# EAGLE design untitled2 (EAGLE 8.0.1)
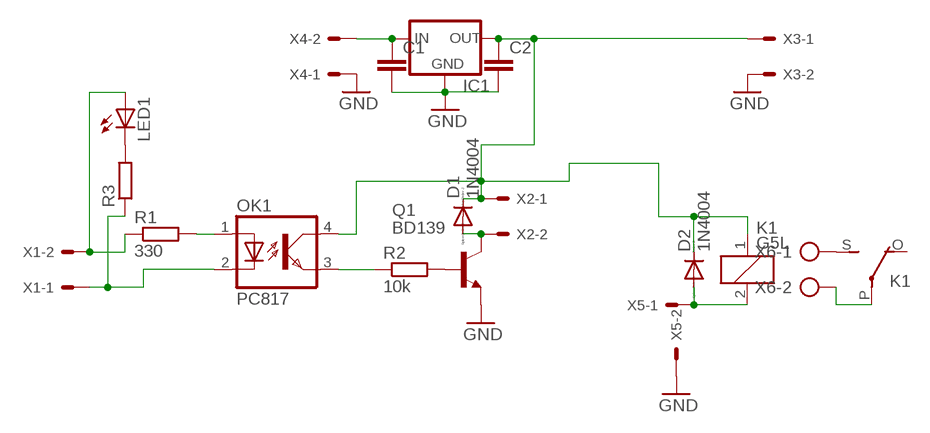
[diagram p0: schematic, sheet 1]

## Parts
C1  C-EU050-024X044  [C050-024X044]
C2  C-EU050-024X044  [C050-024X044]
D1  1N4004  [DO41-10]
D2  1N4004  [DO41-10]
IC1  78XXL  [78XXL]
K1  G5L  [G5LE]
LED1  LED3MM  [LED3MM]
OK1  PC817  [DIL04]
Q1  BD139  [TO126]
R1  330  R-EU_0207/7  [0207/7]
R2  10k  R-EU_0207/10  [0207/10]
R3  R-EU_0207/10  [0207/10]
X1  KK-156-2  [KK-156-2]
X2  KK-156-2  [KK-156-2]
X3  KK-156-2  [KK-156-2]
X4  KK-156-2  [KK-156-2]
X5  KK-156-2  [KK-156-2]
X6  AK300/2  [AK300/2]

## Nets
GND: C1.2 C2.2 IC1.GND Q1.1(E) X3.2 X4.1 X5.2
N$2: OK1.1(A) R1.2
N$3: OK1.2(C) R3.1 X1.1
N$4: Q1.3(B) R2.2
N$5: OK1.3(EMIT) R2.1
N$6: D1.A Q1.2(C) X2.2
N$8: C1.1 IC1.IN X4.2
N$10: C2.1 D1.C D2.C IC1.OUT K1.1 OK1.4(COL) X2.1 X3.1
N$12: D2.A K1.2 X5.1
N$13: K1.S(2:S) X6.1
N$14: K1.P(2:P) X6.2
N$19: LED1.K(C) R3.2
N$42: LED1.A R1.1 X1.2
Unconnected: K1.O(2:O)

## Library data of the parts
C1 C2 = resistor:C-EU: CAPACITOR, European symbol
D1 D2 = diode:1N4004: DIODE
IC1 = v-reg:78XXL: VOLTAGE REGULATOR
K1 = relay:G5L: RELAY 1 x switch, 10 A/120 V AC, 8 A/30 V ADC, Omron; OC_FARNELL: unknown; OC_NEWARK: unknown
LED1 = led:LED: LED
OK1 = optocoupler:PC817: SHARP OPTO COUPLER; MPN: PC817X4J000F; OC_FARNELL: 9707727; OC_NEWARK: 97K7059
Q1 = transistor-npn:BD139*: NPN Transistor
R1-R3 = resistor:R-EU_: RESISTOR, European symbol
X1-X5 = con-molex:KK-156-2: KK 156 HEADER; OC_FARNELL: unknown; OC_NEWARK: unknown
X6 = con-ptr500:AK300/2: CONNECTOR; OC_FARNELL: unknown; OC_NEWARK: unknown

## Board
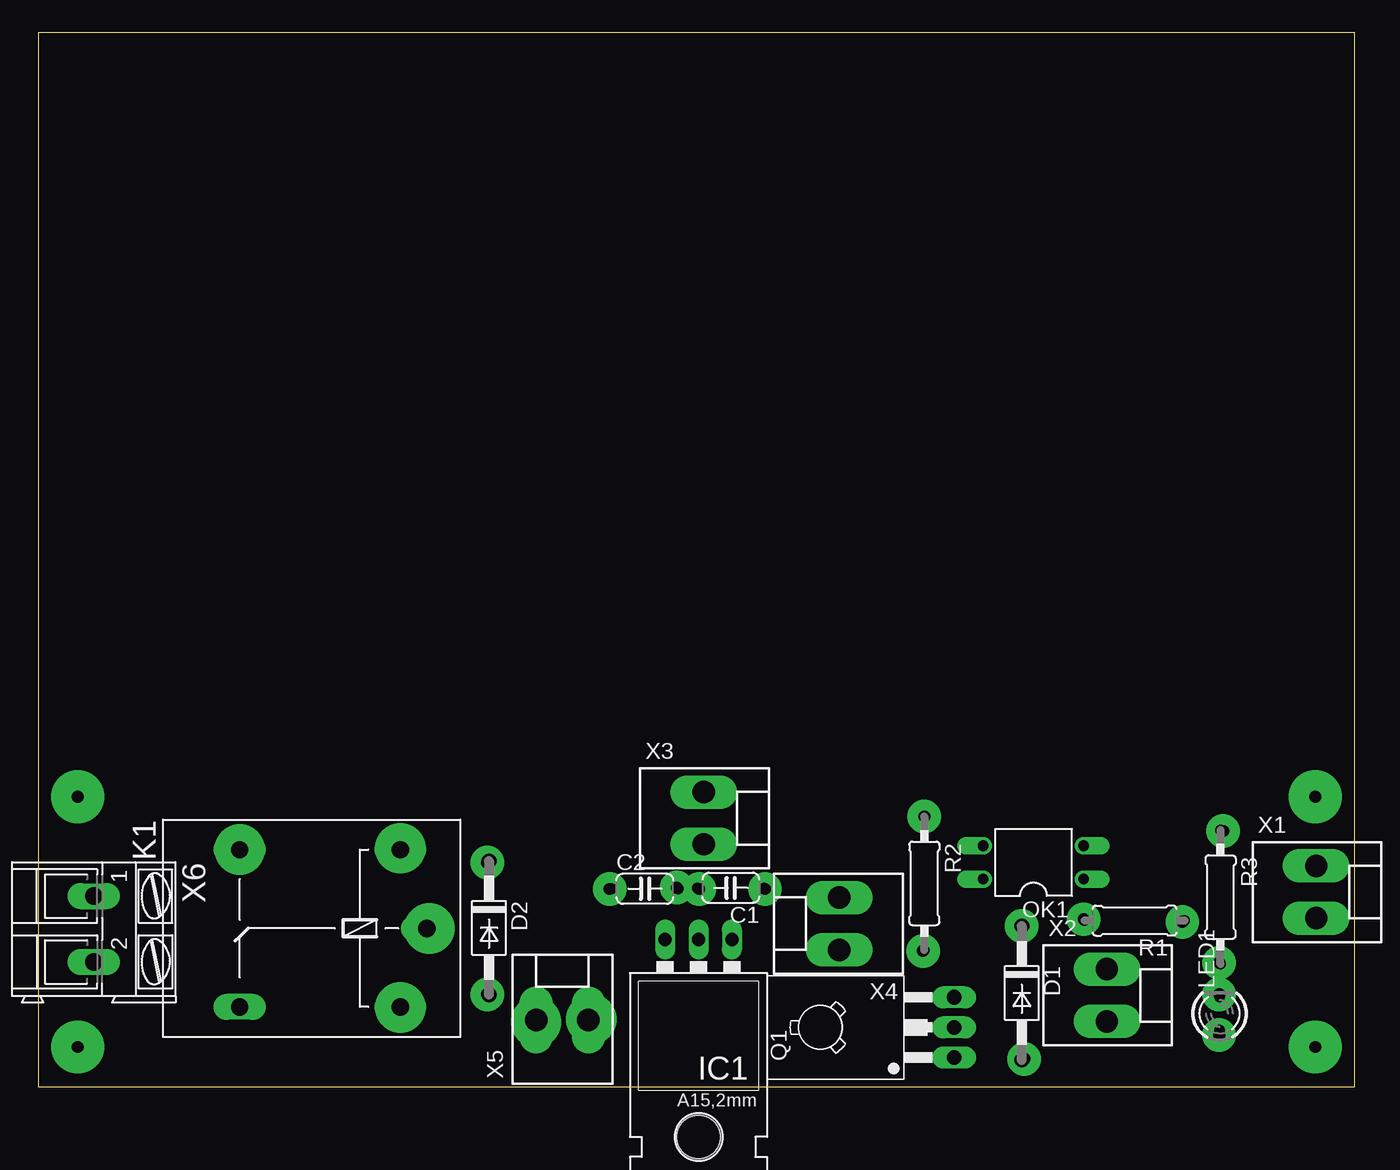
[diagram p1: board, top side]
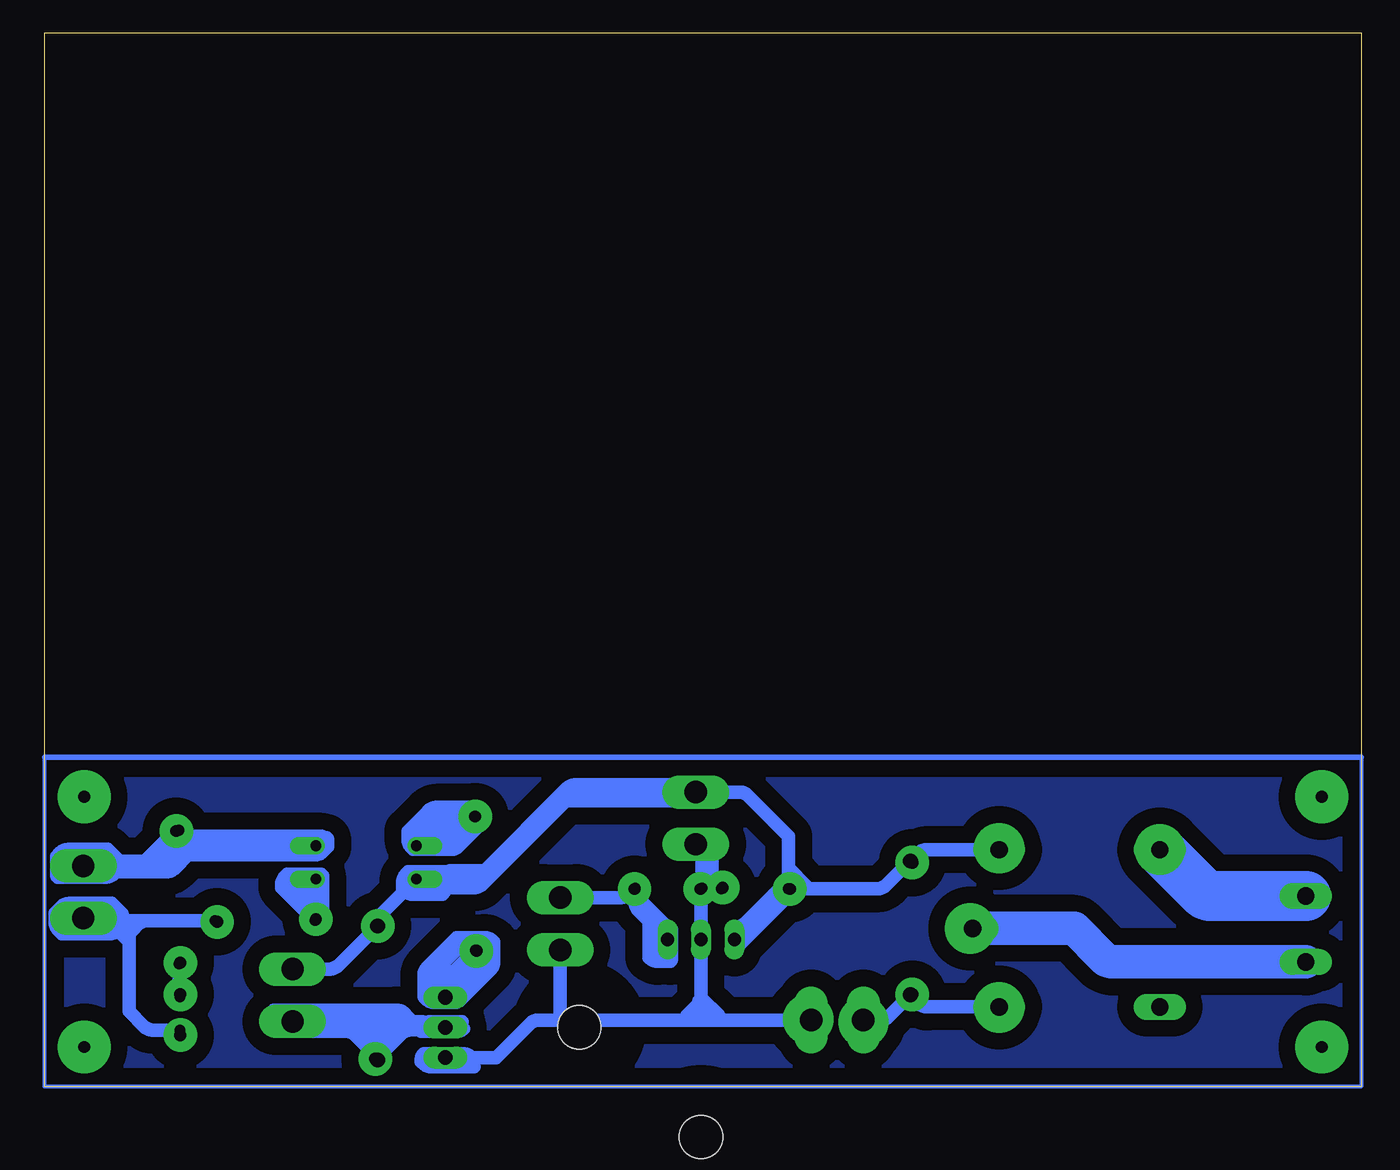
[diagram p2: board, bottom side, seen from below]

Size 100 x 80 mm. Coordinates in mm from the lower left corner, seen from the top.
Outline: 0,0 100,0 100,80 0,80 0,0
Copper layers (1*16): Top 0.035mm / dielectric 1.5mm / Bottom 0.035mm
Design rules "default": minimum track width 10mil, minimum drill 24mil, track to track 8mil, track to pad 8mil, pad to pad 8mil, via to via 8mil, smd to smd 8mil, copper to edge 40mil, drill to drill 8mil, minimum pad ring 10mil, minimum via ring 8mil, stop-mask expansion 4mil, vias tented up to drill 0mil, thermal gap 10mil

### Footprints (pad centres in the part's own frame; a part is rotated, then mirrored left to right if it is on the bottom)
C050-024X044 = drill 0.813 octagon: 1 -2.54,0; 2 2.54,0
DO41-10 = drill 1.118: A 5.08,0; C -5.08,0
78XXL = drill 1.016 long: GND 0,-3.81; IN -2.54,-3.81; OUT 2.54,-3.81 | hole 3.302: 0,11.176
G5LE = drill 1.321 long: 1 -7.493,-5.969; 2 -7.493,5.969; O 4.699,5.969; P -9.525,0; S 4.699,-5.969
LED3MM = drill 0.813 octagon: A -1.27,0; K 1.27,0
DIL04 = drill 0.813 offset: 1 -1.27,-3.81; 2 1.27,-3.81; 3 1.27,3.81; 4 -1.27,3.81
TO126 = drill 1.118 long: 1 -2.286,-5.08; 2 0,-5.08; 3 2.286,-5.08 | hole 3.302: 0,5.08
0207/7 = drill 0.813 octagon: 1 -3.81,0; 2 3.81,0
0207/10 = drill 0.813 octagon: 1 -5.08,0; 2 5.08,0
KK-156-2 = drill 1.7 pad 2.184 long: 1 -1.98,0; 2 1.98,0
AK300/2 = drill 1.321 long: 1 -2.515,0; 2 2.489,0

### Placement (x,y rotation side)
C1  52.61,15.08 180 top
C2  46.07,15.02 0 top
D1  74.71,7.1 270 top
D2  34.24,12.05 270 top
IC1  50.15,7.35 180 top
K1  20,12.01 180 top
LED1  89.73,5.55 90 top
OK1  75.59,17.02 90 top
Q1  64.48,4.49 90 top
R1  83.27,12.6 180 top
R2  67.3,15.43 270 top
R3  89.8,14.38 270 top
X1  97.07,14.77 270 top
X2  81.17,6.93 270 top
X3  50.55,20.38 270 top
X4  60.85,12.36 90 top
X5  39.8,5.05 0 top
X6  4.21,11.95 270 top

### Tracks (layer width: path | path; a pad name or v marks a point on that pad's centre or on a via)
GND
  Bottom 1.016: 50,5.05 X5.2 | 60.7,5.05 50,5.05 | 60.7,5.05 62.44,5.05 arc-45 63.14,4.76 65.7,2.2 Q1.1 arc45 Q1.1 | 50,5.05 arc45 50.15,5.41 IC1.GND 50.15,14.89 arc45 C1.2 | C2.2 49.92,15.02 arc45 C1.2 | C1.2 50.07,17.51 arc-45 50.36,18.21 X3.2 | X4.1 60.85,5.41 arc-45 60.7,5.05
N$1
  pour Bottom (isolate 1.27): 1,24 99,24 99,1 1,1
N$2
  Bottom 1.016: OK1.1 79.4,12.74 arc45 R1.2
N$3
  Bottom 1.016: X1.1 92.92,16.75 arc-45 92.22,17.04 R3.1 88.92,18.58 arc-45 88.22,18.29 OK1.2
N$4
  Bottom 1.016: Q1.3 69.56,7.68 arc45 69.27,8.38 R2.2
N$5
  Bottom 1.016: R2.1 69.68,20.51 arc-45 70.38,20.22 71.5,19.1 71.5,18.97 arc45 OK1.3
N$6
  Bottom 1.016: 74.9,4.49 Q1.2 | 74.9,4.49 81.48,4.49 arc45 81.5,4.5 arc45 81.42,4.71 X2.2 | D1.A 74.71,4.03 arc-45 74.9,4.49
N$7
  Bottom 0.305: 0,25 0,0 100,0 100,25
  Bottom 0.406: 0,25 100,25
N$8
  Bottom 1.016: X4.2 56.3,14.34 arc-45 55.6,14.63 C1.1 55.15,14.03 arc-45 54.86,13.33 IC1.IN
N$9  (via drill 0.9 pad 2.54)
  other vias: 34.1,17
N$10
  Bottom 1.016: K1.1 32.98,17.98 arc-45 33.68,17.69 D2.C 36.06,15.31 arc45 36.76,15.02 C2.1 43.92,14.62 | IC1.OUT arc-45 47.23,11.32 43.92,14.62 | 43.92,14.62 43.79,14.76 arc-45 43.5,15.46 43.5,19 46.57,22.07 arc-45 47.27,22.36 X3.1 60.13,22.36 arc-45 60.83,22.07 67.1,15.8 71.66,15.8 arc-45 OK1.4 74.42,13.11 arc-45 74.71,12.41 D1.C 77.69,9.2 arc45 78.39,8.91 X2.1
N$11  (via drill 0.9 pad 2.54)
  other vias: 34.1,7
N$12
  Bottom 1.016: X5.1 36.57,5.05 arc-45 35.87,5.34 D2.A 33.6,6.33 arc-45 32.9,6.04 K1.2
N$13
  Bottom 3.81: X6.1 11.37,14.46 arc45 12.08,14.76 K1.S
N$14
  Bottom 2.54: X6.2 18.85,9.46 arc45 19.55,9.75 21.8,12 29.5,12 arc45 K1.P
N$15  (via drill 0.9 pad 2.54)
  other vias: 43.4,15
N$16  (via drill 0.9 pad 2.54)
  other vias: 48.5,15.1
N$17  (via drill 0.9 pad 2.54)
  other vias: 50.2,15
N$18  (via drill 0.9 pad 2.54)
  other vias: 55.2,15
N$19
  Bottom 1.016: R3.2 89.8,6.99 arc-45 LED1.K
N$20  (via drill 0.9 pad 2.54)
  other vias: 67.2,10.3
N$21  (via drill 0.9 pad 2.54)
  other vias: 74.7,12.2
N$22  (via drill 0.9 pad 2.54)
  other vias: 74.9,2.1
N$23  (via drill 0.9 pad 2.54)
  other vias: 79.4,12.7
N$24  (via drill 0.9 pad 2.54)
  other vias: 86.9,12.5
N$25  (via drill 0.9 pad 2.54)
  other vias: 89.7,9.4
N$26  (via drill 0.9 pad 2.54)
  other vias: 89.7,7
N$27  (via drill 0.9 pad 2.54)
  other vias: 89.7,3.9
N$28  (via drill 0.9 pad 2.54)
  other vias: 90,19.4
N$29  (via drill 0.9 pad 2.54)
  other vias: 67.3,20.5
N$30  (via drill 0.9 pad 3.81)
  other vias: 27.5,6
N$31  (via drill 0.9 pad 3.81)
  other vias: 29.7,12
N$32  (via drill 0.9 pad 3.81)
  other vias: 27.5,18.1
N$33  (via drill 0.9 pad 3.81)
  other vias: 15.3,18
N$34  (via drill 0.9 pad 3.81)
  other vias: 42,5.1
N$35  (via drill 0.9 pad 3.81)
  other vias: 37.8,4.9
N$36
  Bottom 1.016: 79.2,19 81.6,19 | 81.6,19 arc-90 82,18.6 arc90 81.9,18.5 81.9,17.9 arc-45 81.42,17.7 79.2,17.7 78.87,18.03 arc-45 78.8,18.2 78.8,18.9 arc-45 79.04,19 79.1,19 79.71,18.39 arc45 80.41,18.1 80.5,18.1 | 81.3,18.8 arc45 81.47,18.87 81.6,19 | 81.6,19 88.99,19 arc45 89.69,19.29 89.8,19.4 arc-45 90.31,19.19 92.4,17.1 94.79,17.1 arc-45 95.49,16.81 95.6,16.7 95.6,16.3 90.81,16.3 arc-45 90.11,16.59 89.1,17.6 79.51,17.6 arc-45 78.81,17.89 78.5,18.2 78.5,18.66 arc-45 78.6,18.9 82.39,18.9 arc-45 83.09,18.61 83.9,17.8 88.19,17.8 arc45 88.89,18.09 89,18.2 arc45 89.51,18.41 89.7,18.6 arc45 89.84,18.26 91.4,16.7 arc-45 91.06,16.84 89.8,18.1 89.8,17.4 90.06,17.4 arc-45 90.3,17.3
N$37
  Bottom 1.016: 79,16.1 81.6,16.1 81.71,15.99 arc-45 82,15.29 82,15.1 80.14,13.24 arc45 80,12.9 arc-45 79.9,13.14 79.9,13.8 81.33,15.23 arc45 81.4,15.4 arc45 81.16,15.5 80,15.5 80,14.8 78.97,15.83 arc-45 78.9,16 78.9,12.8
N$38
  Bottom 1.016: 69.6,16.3 72.4,16.3 72.51,16.19 arc-45 72.8,15.49 72.8,15 72.69,14.89 arc-45 71.99,14.6 69.8,14.6 69.79,14.61 arc-45 69.5,15.31 69.5,16.3 70.26,15.54 arc45 70.6,15.4 arc-45 71.08,15.6 72,15.6 arc-45 71.9,15.84 71.9,15.9 arc-45 71.42,15.7 70.4,15.7
N$39
  Bottom 1.016: 70.3,18 69.21,18 arc-45 68.51,18.29 66.7,20.1 arc-45 66.84,20.44 67.6,21.2 70.19,21.2 arc-45 70.89,20.91 72.4,19.4 72.4,18.81 arc-45 72.11,18.11 72,18 70.01,18 arc-45 69.31,18.29 67.9,19.7 68.79,19.7 arc-45 69.49,19.41 70.7,18.2 arc45 71.04,18.34 71.1,18.4 arc45 71.03,18.57 69.3,20.3
N$40
  Bottom 1.016: 94.6,17.4 95.2,18 98.19,18 arc-45 98.89,17.71 99.1,17.5 99.1,16.14 arc-45 99,15.9 95.41,15.9 arc-45 94.71,16.19 94.4,16.5
N$41
  Bottom 1.016: 96.6,17.2 98.06,17.2 arc45 98.3,17.3 98.3,16.9 96.81,16.9 arc-45 96.11,17.19 95.7,17.6 97.09,17.6 arc-45 97.79,17.31 98.4,16.7
N$42
  Bottom 1.016: 94.1,12.9 arc-45 94.24,13.24 94.9,13.9 98.09,13.9 arc-45 98.79,13.61 99.2,13.2 99.2,12.51 arc-45 98.91,11.81 98.7,11.6 95.11,11.6 arc-45 94.41,11.89 94.2,12.1 94.59,12.1 arc45 95.29,12.39 96,13.1 98.06,13.1 arc-45 98.3,13 98.3,12.64 arc-45 98.2,12.4 96.88,12.4 arc-45 96.4,12.6 | 93.9,12.6 R1.1 | 93.9,12.6 96.4,12.6 | 96.4,12.6 96.61,12.6 arc45 X1.2 | LED1.A 91.77,4.28 arc45 92.47,4.57 93.6,5.7 93.6,11.89 arc-45 93.89,12.59 93.9,12.6 | 96.4,12.6 arc45 97.08,12.88 97.1,12.9 95.81,12.9 arc-45 95.11,13.19 94.9,13.4
N$43
  Bottom 1.016: 94.7,11.8 arc45 94.19,11.59 93.7,11.1
N$44
  Bottom 1.016: 92.6,12.5 arc-45 92.77,12.43 93.4,11.8
N$45
  Bottom 1.016: 67.4,1.5 70.59,1.5 arc45 71.29,1.79 71.4,1.9 71.4,2.02 arc45 71.2,2.5 68.31,2.5 arc45 67.61,2.21 67.4,2
N$46
  Bottom 1.016: 68.3,4.9 70.79,4.9 arc-45 71.49,4.61 71.5,4.6 71.5,4.44 arc-45 71.4,4.2 68.68,4.2 arc-45 68.2,4.4
N$47
  Bottom 1.016: 68.7,6.4 70.39,6.4 arc45 71.09,6.69 71.2,6.8 71.2,8.39 arc45 70.91,9.09 68.7,11.3 66.61,11.3 arc45 65.91,11.01 65.9,11 65.9,9.51 arc45 66.19,8.81 68.5,6.5 69.49,6.5 arc45 70.19,6.79 70.6,7.2 70.6,8.09 arc45 70.31,8.79 68.3,10.8 67.31,10.8 arc45 66.61,10.51 66.6,10.5 66.6,9.51 arc45 66.89,8.81 69.1,6.6 69.19,6.6 arc45 69.89,6.89 70.4,7.4 70.4,7.89 arc45 70.11,8.59 70,8.7 68.71,8.7 arc-45 68.01,8.99 67.1,9.9 67.1,9.71 arc45 67.39,9.01 69.2,7.2
N$48
  Bottom 1.016: 82.6,5.8 73.31,5.8 arc45 72.61,5.51 71.8,4.7 71.8,4.54 arc-45 71.7,4.3 72.19,4.3 arc-45 72.89,4.01 74.1,2.8 74.1,3.22 arc45 73.9,3.7 arc45 73.62,4.38 73.1,4.9 81.49,4.9 arc45 82.19,5.19 82.2,5.2 82.2,4.91 arc45 82.49,4.21 82.5,4.2 77.11,4.2 arc45 76.41,3.91 74.7,2.2 74.7,2.79 arc-45 74.99,3.49 75.5,4
N$49
  Bottom 1.016: 71.8,4.9 71.3,4.9
N$50
  Bottom 1.016: 69.6,15.1 67.41,15.1 arc-45 66.71,15.39 60.4,21.7 50.41,21.7 arc-45 49.71,21.99 48.8,22.9 59.69,22.9 arc-45 60.39,22.61 66.6,16.4 69.06,16.4 arc-45 69.3,16.3
N$51
  Bottom 1.016: 52.4,11.9 52.4,9.74 arc45 52.5,9.5 53.39,9.5 arc45 54.09,9.79 54.1,9.8 54.1,12.49 arc-45 54.39,13.19 55.6,14.4 55.41,14.4 arc45 54.71,14.11 52.7,12.1 52.7,10.2 53.36,10.2 arc45 53.6,10.3 53.6,11.16 arc-45 53.7,11.4
N$52
  Bottom 1.016: 47.5,12.1 arc-45 46.82,12.38 44,15.2 arc-45 43.72,14.52 43.6,14.4 47.3,10.7
N$53
  Bottom 1.016: 50.3,6.5 arc45 50.44,6.16 51.2,5.4 49.04,5.4 arc45 48.8,5.3 arc-45 48.87,5.47 50,6.6
N$54
  Bottom 1.016: 42.2,15.3 43.4,16.5
N$55
  Bottom 1.016: 49.3,17.4 49.3,15.68 arc-45 49.1,15.2
N$56  (via drill 0.9 pad 4)
  other vias: 3,22
N$57  (via drill 0.9 pad 4)
  other vias: 3,3
N$58  (via drill 0.9 pad 4)
  other vias: 97,3
N$59  (via drill 0.9 pad 4)
  other vias: 97,22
